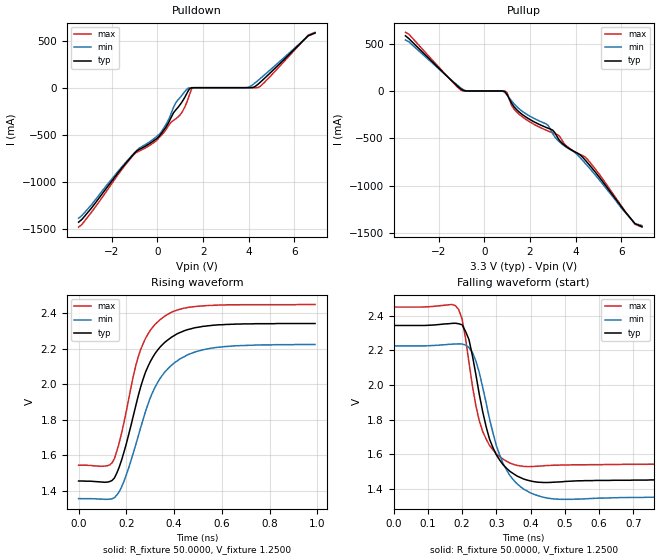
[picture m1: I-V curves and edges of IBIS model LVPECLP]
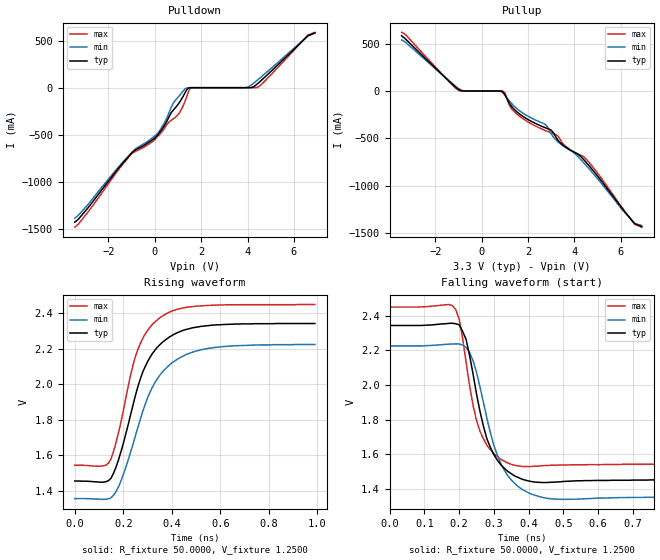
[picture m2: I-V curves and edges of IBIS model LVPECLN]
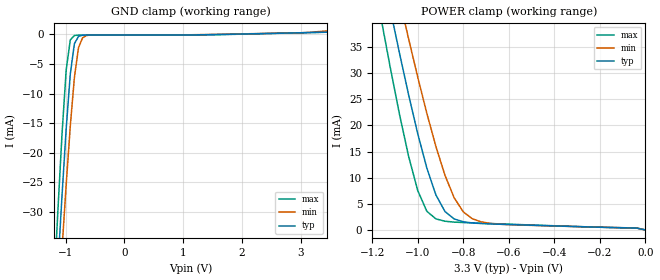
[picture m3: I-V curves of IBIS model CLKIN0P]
|   National Semiconductor Corporation
|   IBIS Model of LMK01020
[IBIS Ver]   3.2
[File name]   lmk01020.ibs
[File Rev]   1.0   | Initial Release
[Notes] Created by Pegah Alavi
   Rev1.0 : Initial Release
[Date]   04/08/2009
[Source]
[Disclaimer]
(C) Copyright National Semiconductor Corporation 2009
   All rights reserved
National Semiconductor Corporation hereby grants the
user of this IBIS model a non-exclusive, nontransferable
license to use this IBIS model under the following terms.
Before using this IBIS model, the user should read this
license.  If the user does not accept these terms,  the
IBIS model should be returned to National within 30 days.
The user is granted this license only to use the
IBIS model and is not granted rights to sell, load, rent,
lease or license the IBIS model in whole or in part, or in
modified form to anyone other than user. User may modify
the IBIS model to suit its specific applications but rights
to derivative works and such modifications shall belong to
National.
This IBIS model is provided on an "AS IS" basis and
National makes absolutely no warranty with respect to the
information contained herein.NATIONAL DISCLAIMS AND CUSTOMER
WAIVES ALL WARRANTIES, EXPRESS OR IMPLIED, INCLUDING
WARRANTIES OF MERCHANTABILITY OR FITNESS FOR A PARTICULAR
PURPOSE. The entire risk as to quality and performance is
with the Customer. ACCORDINGLY, IN NO EVENT SHALL THE
COMPANY BE LIABLE FOR ANY DAMAGES, WHETHER IN CONTRACT OR
TORT,INCLUDING ANY LOST PROFITS OR OTHER INCIDENTAL,
CONSEQUENTIAL, EXEMPLARY, OR PUNITIVE DAMAGES ARISING OUT
OF THE USE OR APPLICATION OF THE IBIS model provided in
this package.Further, National reserves the right to make
changes without notice to any product herein to improve
reliability, function, or design. National does not convey
any license under patent rights or any other intellectual
property rights, including those of third parties.
National is not obligated to provide maintenance or support
for the licensed IBIS model.
[Copyright]  Copyright 2009, National Semiconductor, All Rights Reserved
[Component]  LMK01020
[Manufacturer]  National Semiconductor Corp
[Package]
|   typ   min   max
R_pkg   0.693   0.432   0.954
L_pkg   1.875nH   1.120nH   2.630nH
C_pkg   0.046pF   0.037pF   0.055pF
[Pin]   signal_name   model_name   R_pin   L_pin   C_pin
1   GND   GND   0.856   2.350nH   0.055pF
2   NC   NC   0.769   2.080nH   0.042pF
3   Vcc1   POWER   0.732   1.960nH   0.040pF
4   CLKuWire   NC   0.71   1.890nH   0.040pF
5   DATAuWire   NC   0.701   1.860nH   0.040pF
6   LEuWire   NC   0.711   1.890nH   0.039pF
7   NC   NC   0.712   1.850nH   0.045pF
8   VCC2   POWER   0.806   2.150nH   0.040pF
9   NC   NC   0.736   1.850nH   0.042pF
10   NC   NC   0.718   1.910nH   0.041pF
11   GOE   NC   0.719   1.940nH   0.041pF
12   TEST   NC   0.751   2.080nH   0.055pF
13   VCC3   POWER   0.736   2.070nH   0.051pF
14   CLKout0   LVPECLP   0.715   1.970nH   0.040pF
15   CLKout0*   LVPECLN   0.637   1.730nH   0.039pF
16   VCC4   POWER   0.601   1.620nH   0.038pF
17   CLKout1   LVPECLP   0.533   1.410nH   0.037pF
18   CLKout1*   LVPECLN   0.475   1.240nH   0.037pF
19   VCC5   POWER   0.447   1.160nH   0.037pF
20   CLKout2   LVPECLP   0.432   1.120nH   0.038pF
21   CLKout2*   LVPECLN   0.442   1.140nH   0.038pF
22   VCC6   POWER   0.465   1.220nH   0.038pF
23   CLKout3   LVPECLP   0.488   1.300nH   0.039pF
24   CLKout3*   LVPECLN   0.542   1.490nH   0.050pF
25   GND   GND   0.666   1.850nH   0.053pF
26   VCC7   POWER   0.580   1.550nH   0.041pF
27   SYNC*   NC   0.508   1.330nH   0.039pF
28   CLKIN0   CLKIN0P   0.469   1.220nH   0.039pF
29   CLKIN0*   CLKIN0N   0.447   1.160nH   0.039pF
30   VCC8   POWER   0.442   1.130nH   0.038pF
31   VCC9   POWER   0.467   1.160nH   0.040pF
32   NC   NC   0.461   1.200nH   0.039pF
33   VCC10   POWER   0.488   1.270nH   0.039pF
34   CLKIN1   CLKIN1P   0.526   1.390nH   0.039pF
35   CLKIN1*   CLKIN1N   0.593   1.580nH   0.041pF
36   BIAS   POWER   0.658   1.810nH   0.053pF
37   VCC11   POWER   0.677   1.880nH   0.051pF
38   CLKout4   LVPECLP   0.666   1.800nH   0.040pF
39   CLKout4*   LVPECLN   0.630   1.670nH   0.038pF
40   VCC12   POWER   0.613   1.620nH   0.039pF
41   CLKout5   LVPECLP   0.611   1.610nH   0.038pF
42   CLKout5*   LVPECLN   0.634   1.680nH   0.038pF
43   VCC13   POWER   0.663   1.760nH   0.038pF
44   CLKout6   LVPECLP   0.701   1.870nH   0.038pF
45   CLKout6*   LVPECLN   0.765   2.040nH   0.038pF
46   VCC14   POWER   0.817   2.190nH   0.039pF
47   CLKout7   LVPECLP   0.874   2.370nH   0.039pF
48   CLKout7*   LVPECLN   0.954   2.630nH   0.051pF
49   DAP   NC
[Diff pin]  inv_pin  vdiff  tdelay_typ  tdelay_min  tdelay_max
14 15   0.0V   0.0s   0.0s   0.0s
17 18   0.0V   0.0s   0.0s   0.0s
20 21   0.0V   0.0s   0.0s   0.0s
23 24   0.0V   0.0s   0.0s   0.0s
28 29   200mV   0.0s   0.0s   0.0s
34 35   200mV   0.0s   0.0s   0.0s
38 39   0.0V   0.0s   0.0s   0.0s
41 42   0.0V   0.0s   0.0s   0.0s
44 45   0.0V   0.0s   0.0s   0.0s
47 48   0.0V   0.0s   0.0s   0.0s
[Define Package Model]  48_LLP_for_LMK01020ISQ_AC_model_at_5_GHz
[Manufacturer]   National Semiconductor Corporation
[OEM]   NA
[Description]   48 LLP for LMK01020ISQ, full model
[Number Of Pins]   49
[Pin Numbers]
   1   |   1 = 1
   2   |   2 = 2
   3   |   3 = 3
   4   |   4 = 4
   5   |   5 = 5
   6   |   6 = 6
   7   |   7 = 7
   8   |   8 = 8
   9   |   9 = 9
  10   |  10 = 10
  11   |  11 = 11
  12   |  12 = 12
  13   |  13 = 13
  14   |  14 = 14
  15   |  15 = 15
  16   |  16 = 16
  17   |  17 = 17
  18   |  18 = 18
  19   |  19 = 19
  20   |  20 = 20
  21   |  21 = 21
  22   |  22 = 22
  23   |  23 = 23
  24   |  24 = 24
  25   |  25 = 25
  26   |  26 = 26
  27   |  27 = 27
  28   |  28 = 28
  29   |  29 = 29
  30   |  30 = 30
  31   |  31 = 31
  32   |  32 = 32
  33   |  33 = 33
  34   |  34 = 34
  35   |  35 = 35
  36   |  36 = 36
  37   |  37 = 37
  38   |  38 = 38
  39   |  39 = 39
  40   |  40 = 40
  41   |  41 = 41
  42   |  42 = 42
  43   |  43 = 43
  44   |  44 = 44
  45   |  45 = 45
  46   |  46 = 46
  47   |  47 = 47
  48   |  48 = 48
  49   |  49 = DAP
[Model Data]
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[End Model Data]
[End Package Model]
| Models and submodels in the file (6): LVPECLP (Output), LVPECLN (Output), CLKIN0P (Input), CLKIN0N (Input), CLKIN1P (Input), CLKIN1N (Input)
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|   Model LVPECLP
[Model]  LVPECLP
Model_type Output
Polarity   Non-Inverting
Vmeas =  1.9400V
Rref =   50.0000
Vref =   1.2500V
C_comp   1.1000pF   1.1000pF   1.100pF
[Temperature Range]   25.0000   85.0000   -40.0000
[Voltage Range]   3.3000V   3.1500V   3.4500V
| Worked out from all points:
|   slope of the pulldown table from 0 to 0.495 V, typ, clamps not added: 2.95 ohm
|   rising waveform, R_fixture 50.0000, V_fixture 1.2500: 20-80 % time 123ps typ, 140ps min, 104ps max; typ from 1.46 V to 2.34 V
|   falling waveform, R_fixture 50.0000, V_fixture 1.2500: 20-80 % time 61.3ps typ, 72ps min, 51.6ps max; typ from 2.34 V to 1.45 V
[Pulldown]
|Voltage   I(typ)   I(min)   I(max)
-3.45V    -1.429A    -1.387A    -1.482A
-1.1V     -722.9mA   -716.3mA   -729.3mA
100mV     -509.2mA   -491.3mA   -523.3mA
400mV     -409mA     -379.8mA   -437mA
800mV     -237.4mA   -162.8mA   -331.3mA
1V        -178mA     -102.2mA   -287.5mA
1.2V      -101.2mA   -41.1mA    -204.8mA
1.5V      -613.3uA   -58.5uA    -11.3mA
3.9V      173.5nA    754.6uA    57.2pA
4.4V      36.18mA    76.19mA    1.372mA
6.6V      551.6mA    550.5mA    558.3mA
6.9V      581.6mA    580.5mA    588.3mA
[Pullup]
|Voltage   I(typ)   I(min)   I(max)
-3.45V    581.6mA    537.7mA    618.2mA
-1V       16.83mA    27.74mA    5.801mA
900mV     -5.507mA   -15.29mA   -325.7uA
1V        -38.16mA   -43.45mA   -19.47mA
1.2V      -130.1mA   -105.9mA   -154.5mA
1.5V      -215.9mA   -182.5mA   -239.6mA
2.8V      -392.6mA   -364.2mA   -422.4mA
3.2V      -486.7mA   -515.5mA   -460.3mA
3.6V      -587.8mA   -594.2mA   -579.3mA
4.5V      -751.4mA   -783.9mA   -716.1mA
6.6V      -1.398A    -1.397A    -1.405A
6.9V      -1.428A    -1.417A    -1.435A
[Ramp]
| variable   typ   min   max
dV/dt_r  0.5335/0.1232n   0.5233/0.1420n   0.5443/0.1040n
dV/dt_f  0.5335/0.0610n   0.5220/0.0720n   0.5452/0.0514n
R_load = 50.0000
[Rising Waveform]
R_fixture= 50.0000
V_fixture= 1.2500
V_fixture_min= 1.2300
V_fixture_max= 1.2700
|time   V(typ)   V(min)   V(max)
0s        1.455V     1.356V     1.544V
140ps     1.458V     1.355V     1.557V
190ps     1.618V     1.454V     1.785V
230ps     1.827V     1.617V     2.051V
260ps     1.985V     1.756V     2.195V
300ps     2.126V     1.923V     2.302V
360ps     2.234V     2.067V     2.382V
430ps     2.293V     2.146V     2.423V
550ps     2.329V     2.201V     2.443V
990ps     2.341V     2.223V     2.448V
[Falling Waveform]
R_fixture= 50.0000
V_fixture= 1.2500
V_fixture_min= 1.2300
V_fixture_max= 1.2700
|time   V(typ)   V(min)   V(max)
0s        2.343V     2.225V     2.449V
170ps     2.355V     2.235V     2.464V
200ps     2.347V     2.236V     2.38V
220ps     2.262V     2.216V     2.131V
240ps     2.063V     2.14V      1.883V
260ps     1.847V     1.988V     1.732V
300ps     1.597V     1.65V      1.603V
340ps     1.501V     1.476V     1.549V
470ps     1.439V     1.342V     1.537V
990ps     1.454V     1.355V     1.544V
|   Model LVPECLN
[Model]  LVPECLN
Model_type Output
Polarity   Inverting
Vmeas =  1.9400V
Rref =   50.0000
Vref =   1.2500V
C_comp   1.1000pF   1.1000pF   1.1000pF
[Temperature Range]   25.0000   85.0000   -40.0000
[Voltage Range]   3.3000V   3.1500V   3.4500V
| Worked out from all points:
|   slope of the pulldown table from 0 to 0.495 V, typ, clamps not added: 2.95 ohm
|   rising waveform, R_fixture 50.0000, V_fixture 1.2500: 20-80 % time 123ps typ, 140ps min, 104ps max; typ from 1.46 V to 2.34 V
|   falling waveform, R_fixture 50.0000, V_fixture 1.2500: 20-80 % time 61.3ps typ, 72ps min, 51.6ps max; typ from 2.34 V to 1.45 V
[Pulldown]
|Voltage   I(typ)   I(min)   I(max)
-3.45V    -1.429A    -1.387A    -1.482A
-1.1V     -722.9mA   -716.3mA   -729.3mA
100mV     -509.2mA   -491.3mA   -523.3mA
400mV     -409mA     -379.8mA   -437mA
800mV     -237.4mA   -162.8mA   -331.3mA
1V        -178mA     -102.2mA   -287.5mA
1.2V      -101.2mA   -41.1mA    -204.8mA
1.5V      -613.3uA   -58.5uA    -11.3mA
3.9V      173.5nA    754.6uA    57.2pA
4.4V      36.18mA    76.19mA    1.372mA
6.6V      551.6mA    550.5mA    558.3mA
6.9V      581.6mA    580.5mA    588.3mA
[Pullup]
|Voltage   I(typ)   I(min)   I(max)
-3.45V    581.6mA    537.7mA    618.2mA
-1V       16.83mA    27.74mA    5.801mA
900mV     -5.507mA   -15.29mA   -325.7uA
1V        -38.16mA   -43.45mA   -19.47mA
1.2V      -130.1mA   -105.9mA   -154.5mA
1.5V      -215.9mA   -182.5mA   -239.6mA
2.8V      -392.6mA   -364.2mA   -422.4mA
3.2V      -486.7mA   -515.5mA   -460.3mA
3.6V      -587.8mA   -594.2mA   -579.3mA
4.5V      -751.4mA   -783.9mA   -716.1mA
6.6V      -1.398A    -1.397A    -1.405A
6.9V      -1.428A    -1.417A    -1.435A
[Ramp]
| variable   typ   min   max
dV/dt_r  0.5335/0.1232n   0.5233/0.1420n   0.5443/0.1040n
dV/dt_f  0.5335/0.0610n   0.5220/0.0720n   0.5452/0.0514n
R_load = 50.0000
[Rising Waveform]
R_fixture= 50.0000
V_fixture= 1.2500
V_fixture_min= 1.2300
V_fixture_max= 1.2700
|time   V(typ)   V(min)   V(max)
0s        1.455V     1.356V     1.544V
140ps     1.458V     1.355V     1.557V
190ps     1.618V     1.454V     1.785V
230ps     1.827V     1.617V     2.051V
260ps     1.985V     1.756V     2.195V
300ps     2.126V     1.923V     2.302V
360ps     2.234V     2.067V     2.382V
430ps     2.293V     2.146V     2.423V
550ps     2.329V     2.201V     2.443V
990ps     2.341V     2.223V     2.448V
[Falling Waveform]
R_fixture= 50.0000
V_fixture= 1.2500
V_fixture_min= 1.2300
V_fixture_max= 1.2700
|time   V(typ)   V(min)   V(max)
0s        2.343V     2.225V     2.449V
170ps     2.355V     2.235V     2.464V
200ps     2.347V     2.236V     2.38V
220ps     2.262V     2.216V     2.131V
240ps     2.063V     2.14V      1.883V
260ps     1.847V     1.988V     1.732V
300ps     1.597V     1.65V      1.603V
340ps     1.501V     1.476V     1.549V
470ps     1.439V     1.342V     1.537V
990ps     1.454V     1.355V     1.544V
|   Model CLKIN0P
[Model]  CLKIN0P
Model_type Input
Polarity   Non-Inverting
Vinl =   1.5300V
Vinh =   1.7300V
C_comp   0.6pF   0.6pF   0.6pF
[Temperature Range]   25.0000   85.0000   -40.0000
[Voltage Range]   3.3000V   3.1500V   3.4500V
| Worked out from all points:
|   GND clamp passes 1 mA (typ) near -0.82 V on its own axis
|   POWER clamp passes 1 mA (typ) near -0.57 V on its own axis
[GND_clamp]
|Voltage   I(typ)   I(min)   I(max)
-3.45V    -488.6mA   -451mA     -506.6mA
-1.2V     -51.66mA   -58.95mA   -43.37mA
-1.13V    -39.16mA   -47.42mA   -29.63mA
-1.06V    -27.13mA   -36.19mA   -16.75mA
-990mV    -15.98mA   -25.44mA   -6.053mA
-920mV    -6.721mA   -15.53mA   -930.4uA
-850mV    -1.576mA   -7.276mA   -176.4uA
-780mV    -328.7uA   -2.224mA   -115.1uA
-710mV    -121.2uA   -560.8uA   -112.7uA
-640mV    -99.89uA   -172.9uA   -112.6uA
2.3V      134.7uA    149.3uA    118.3uA
3.45V     380.2uA    588uA      374uA
[POWER_clamp]
|Voltage   I(typ)   I(min)   I(max)
-3.45V    578.6mA    549mA      626.7mA
-1.16V    50.67mA    59.87mA    40.27mA
-1.12V    42.13mA    51.94mA    30.97mA
-1.08V    33.82mA    44.16mA    22.13mA
-1.04V    25.86mA    36.58mA    14.09mA
-1V       18.44mA    29.27mA    7.547mA
-960mV    11.86mA    22.33mA    3.579mA
-920mV    6.689mA    15.96mA    2.119mA
-880mV    3.513mA    10.43mA    1.67mA
-800mV    1.572mA    3.473mA    1.423mA
-680mV    1.155mA    1.25mA     1.23mA
0V        350.2pA    342.7pA    390.5pA
